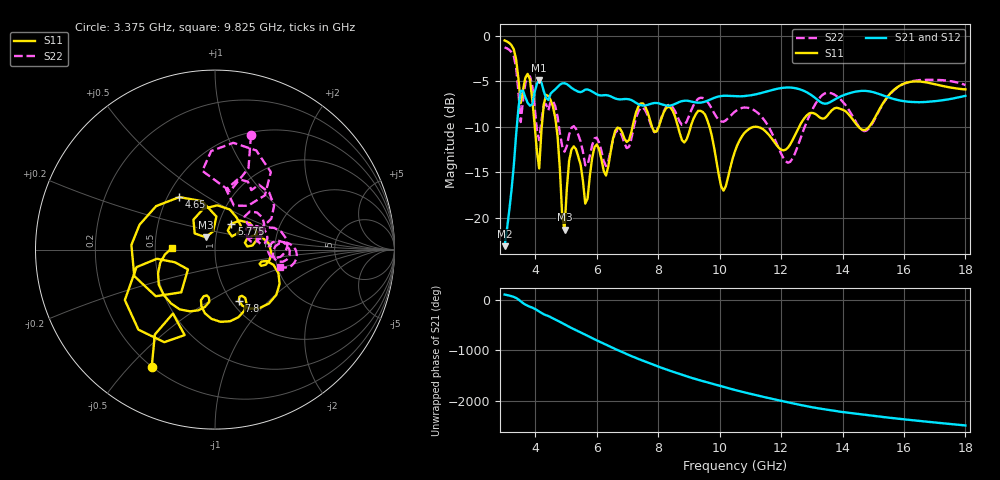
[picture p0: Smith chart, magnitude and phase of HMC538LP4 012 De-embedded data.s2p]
! Chelmsford, MA 01824
! http://www.hittite.com
! Tel: 978-250-3343
! Fax: 978-250-3373
! Device  :  HMC538LP4
! Description:  600 Analog Phase Shifter
! Frequency  :  6.0 GHz - 15.0 GHz
! Package  :  LP4  - 4x4 mm Quad Flatpack No-Lead (QFN) Plastic Package: 24 pin
! Ports  :  2 RF, 1 DC
!  Pin  3  = Rfin  = Port 1
!  Pin  16  = Rfout = Port 2
!  pin  21  = vCTL
! Voltages:  VCTL  = 0 to 5.0 Volts
! Currents :  Vb(V)  Vd(V)  Ib(mA)  Id(mA)
!  0.00  1.20  0.000000	0.489601
! Data:  The device was measured on evaluation board 111296-1.
!  Data was collected using a calibrated network analyzer.
!  The evaluation circuit board was modeled and simulated.This was use
!  to removed the evaluation board circuit from the measured data.
!  The reference plane is the center of the package pin.
! Misc:  Lot #
!Date Measured:  03 - 11 -2009
! Date:  03 - 17 -2009
! Note:
!  Hittite Microwave supplies this data as a sample of measured data at the
!  package pin for this package product.  Your particular data for this product
!  may vary.
!  Data was taken at 25 degrees C.
!  Hittite Microwave reserves the right to change this data at anytime.
# MHz S MA R 50
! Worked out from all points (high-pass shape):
!   201 points, 3 GHz to 18 GHz, reference 50 ohm
!   highest |S21| = -4.85 dB at 4.125 GHz (marker M1); lowest = -23.1 dB at 3 GHz (marker M2)
!   |S21| within 3 dB of the highest: 3.455 GHz to end of sweep
!   lowest |S11| = -21.3 dB at 4.95 GHz (marker M3), VSWR 1.19, Z = 44.7 + j6.2 ohm
!   |S11| at or under -10 dB: 4.686 GHz to 7.164 GHz (2.478 GHz wide, 41.8 % of centre); 9.671 GHz to 11.15 GHz (1.476 GHz wide, 14.2 % of centre); 11.19 GHz to 12.59 GHz (1.396 GHz wide, 11.7 % of centre)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
!   |S22| runs from -14.3 to -1.3 dB; largest |S21 - S12| = 0.0013
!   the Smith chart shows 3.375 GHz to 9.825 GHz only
!   S11 on the Smith chart (normalised r, x): 3.375 GHz: 0.20, -0.58; 4.65 GHz: 0.57, +0.38; 5.775 GHz: 1.15, +0.34; 7.8 GHz: 1.08, -0.68; 9.825 GHz: 0.61, +0.01
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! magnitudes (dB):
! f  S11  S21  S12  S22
! 3 GHz  -0.5  -23.1  -23.1  -1.3
! 3.375 GHz  -2.6  -10.9  -10.9  -3.5
! 3.525 GHz  -7.4  -6.1  -6.1  -9.5
! 3.825 GHz  -4.8  -7.7  -7.7  -4.5
! 4.125 GHz  -14.6  -4.9  -4.9  -11.5
! 4.35 GHz  -6.5  -6.8  -6.8  -7.5
! 4.65 GHz  -9.0  -5.9  -5.9  -7.8
! 4.95 GHz  -21.3  -5.2  -5.2  -12.7
! 5.175 GHz  -12.5  -5.7  -5.7  -10.1
! 5.55 GHz  -15.9  -6.1  -6.1  -12.7
! 5.775 GHz  -15.4  -6.0  -6.0  -13.2
! 7.425 GHz  -7.4  -7.6  -7.6  -7.9
! 7.8 GHz  -10.0  -7.4  -7.4  -10.2
! 8.025 GHz  -9.9  -7.4  -7.4  -9.8
! 9.825 GHz  -12.4  -6.8  -6.8  -8.5
! 10.12 GHz  -17.0  -6.6  -6.6  -9.4
! 10.5 GHz  -12.7  -6.6  -6.6  -8.3
! 12.22 GHz  -12.3  -5.7  -5.7  -14.0
! 13.05 GHz  -8.5  -6.7  -6.7  -7.9
! 14.7 GHz  -10.4  -6.0  -6.1  -10.5
! 15.53 GHz  -6.5  -6.8  -6.8  -6.5
! 18 GHz  -5.9  -6.6  -6.6  -5.4
